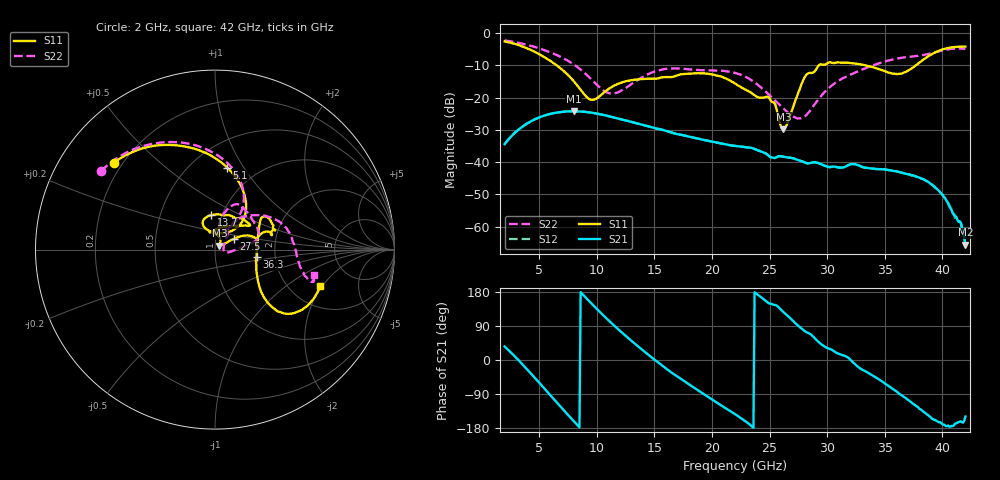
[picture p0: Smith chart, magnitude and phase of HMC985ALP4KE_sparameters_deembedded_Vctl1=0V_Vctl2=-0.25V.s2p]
!s2p File: Measurements: S11, S21, S12, S22
# GHz S dB R 50.0
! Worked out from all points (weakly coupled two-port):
!   401 points, 2 GHz to 42 GHz, reference 50 ohm
!   highest |S21| = -24.21 dB at 8 GHz (marker M1); lowest = -65.5 dB at 42 GHz (marker M2)
!   lowest |S11| = -29.8 dB at 26.2 GHz (marker M3), VSWR 1.07, Z = 52.5 + j2.21 ohm
!   |S11| at or under -10 dB: 6.53 GHz to 29.27 GHz (22.75 GHz wide, 127 % of centre); 33.34 GHz to 37.69 GHz (4.349 GHz wide, 12.2 % of centre)
!   |S22| runs from -26.4 to -2.3 dB; largest |S21 - S12| = 0.00017
!   S11 on the Smith chart (normalised r, x): 2 GHz: 0.17, +0.36; 5.1 GHz: 0.73, +0.85; 13.7 GHz: 0.89, +0.35; 27.5 GHz: 1.22, +0.15; 36.3 GHz: 1.59, -0.14; 42 GHz: 2.91, -1.91
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2  -2.57 139.4  -34.39 35.7  -34.40 35.6  -2.27 145.4
3.5  -4.07 111.5  -29.10 -10.0  -29.11 -10.0  -3.24 121.6
5.1  -6.70 81.5  -25.98 -63.3  -25.98 -63.3  -4.83 97.3
8  -14.88 44.9  -24.21 -161.4  -24.22 -161.4  -9.68 60.6
8.7  -18.04 51.5  -24.31 175.8  -24.32 175.8  -11.59 55.7
9.7  -20.67 87.1  -24.73 144.1  -24.73 144.1  -14.92 54.2
11.2  -16.89 115.7  -25.88 99.4  -25.88 99.5  -18.69 69.7
13.7  -14.29 96.7  -28.16 33.0  -28.16 33.0  -14.17 77.4
15.4  -13.94 73.0  -29.71 -7.9  -29.71 -7.9  -11.49 68.3
19.4  -12.51 34.7  -33.17 -92.2  -33.17 -92.2  -11.52 34.5
22  -15.57 52.2  -34.95 -142.7  -34.93 -142.6  -12.30 13.9
25  -20.23 97.6  -38.22 148.9  -38.25 148.9  -19.25 -2.2
26.2  -29.81 40.7  -38.29 126.4  -38.30 126.5  -23.36 -13.7
27.5  -18.42 29.5  -39.32 90.1  -39.34 90.3  -26.40 -1.6
28.1  -13.36 20.7  -40.16 75.3  -40.11 75.5  -25.68 19.6
28.7  -12.32 12.8  -40.07 64.4  -40.09 63.9  -23.14 37.0
31.1  -9.13 24.1  -41.67 15.2  -41.66 15.4  -14.51 55.4
35.4  -12.27 12.4  -42.49 -70.2  -42.47 -70.3  -8.42 25.8
36.3  -12.57 -10.1  -43.06 -89.9  -43.08 -89.7  -7.74 18.0
39.9  -5.17 -40.4  -49.74 -166.4  -49.71 -167.1  -5.45 -16.9
41.5  -4.18 -23.0  -58.31 -162.7  -58.52 -164.7  -4.75 -17.4
42  -4.14 -19.0  -65.53 -149.3  -66.02 -152.4  -4.90 -14.6
